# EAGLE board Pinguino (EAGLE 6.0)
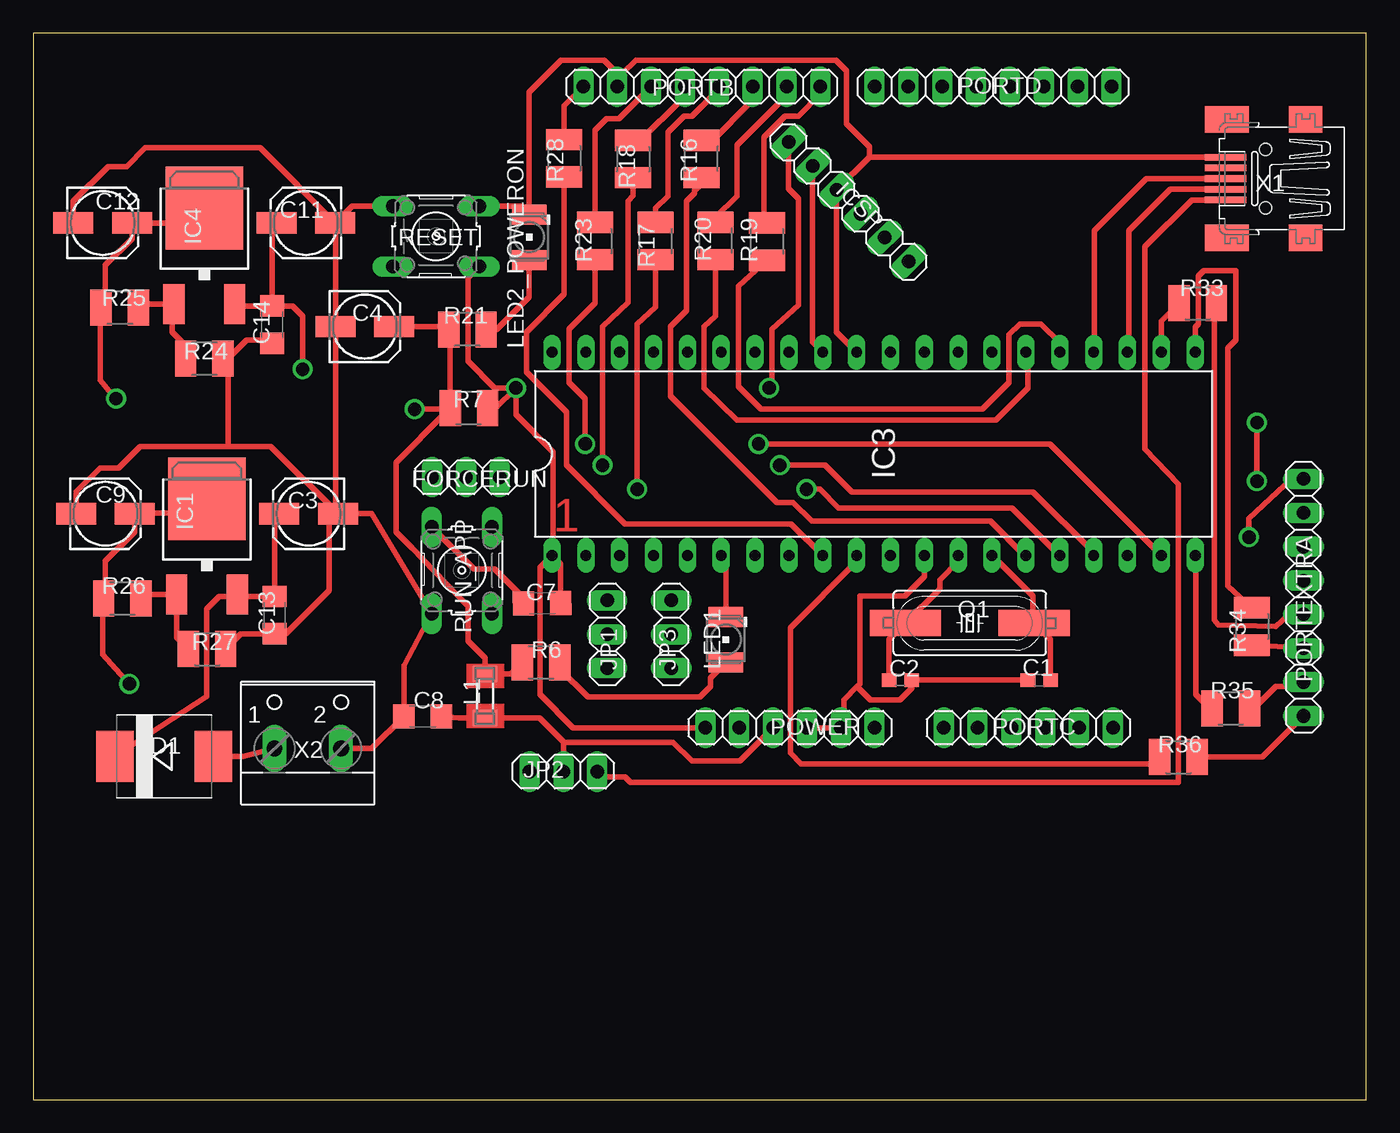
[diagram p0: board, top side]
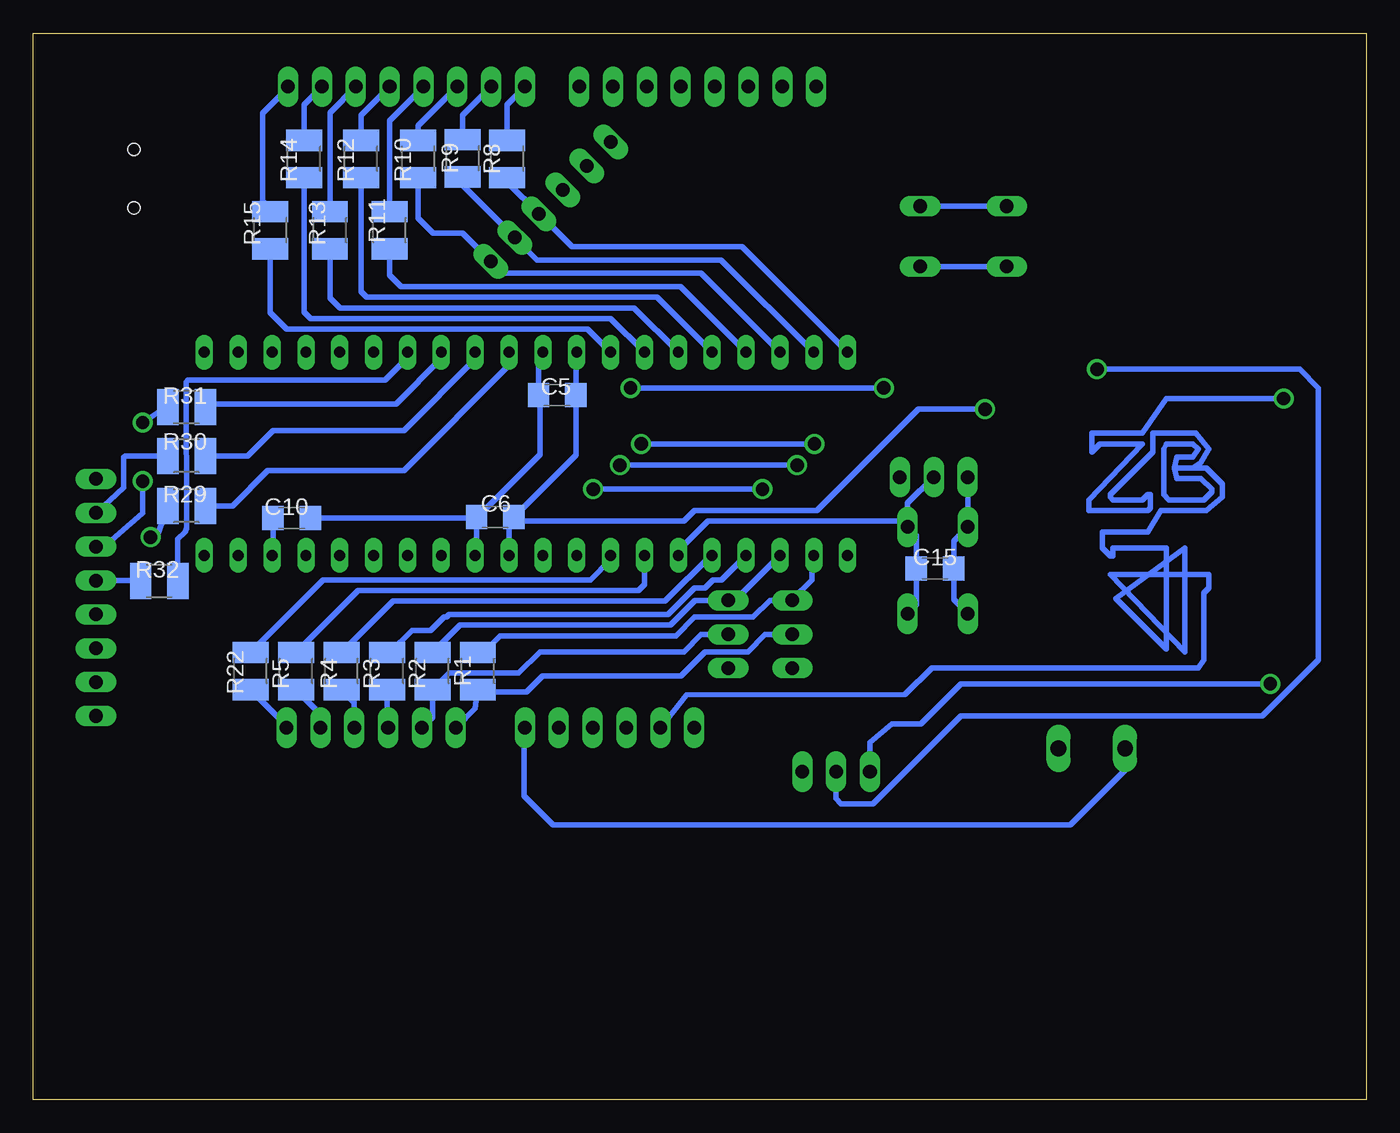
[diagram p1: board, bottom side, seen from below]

Size 100 x 80 mm. Coordinates in mm from the lower left corner, seen from the top.
Outline: 0,0 100,0 100,80 0,80 0,0
Copper layers (1*16): Top 0.035mm / dielectric 1.5mm / Bottom 0.035mm
Design rules: minimum track width 10mil, minimum drill 24mil, track to track 8mil, track to pad 8mil, pad to pad 8mil, via to via 8mil, smd to smd 8mil, copper to edge 40mil, drill to drill 8mil, minimum pad ring 10mil, minimum via ring 8mil, stop-mask expansion 4mil, vias tented up to drill 0mil, thermal gap 10mil

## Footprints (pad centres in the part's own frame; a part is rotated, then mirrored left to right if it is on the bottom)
C0603 = smd 1.1 x 1: 1 -0.85,0; 2 0.85,0
153CLV-0505 = smd 3 x 1.6: + 2.2,0; - -2.2,0
C1206 = smd 1.6 x 1.8: 1 -1.4,0; 2 1.4,0
SMC = smd 2.8 x 3.8: A 3.7,0; C -3.7,0
1X03 = drill 1.016 long: 1 -2.54,0; 2 0,0; 3 2.54,0
DPACK = smd 1.6 x 3: 1 -2.28,-4.8; 3 2.28,-4.8 | smd 5.8 x 6.2: 4 0,2.38
DIL40 = drill 0.813 long: 1 -24.13,-7.62; 2 -21.59,-7.62; 3 -19.05,-7.62; 4 -16.51,-7.62; 5 -13.97,-7.62; 6 -11.43,-7.62; 7 -8.89,-7.62; 8 -6.35,-7.62; 9 -3.81,-7.62; 10 -1.27,-7.62; 11 1.27,-7.62; 12 3.81,-7.62; 13 6.35,-7.62; 14 8.89,-7.62; 15 11.43,-7.62; 16 13.97,-7.62; 17 16.51,-7.62; 18 19.05,-7.62; 19 21.59,-7.62; 20 24.13,-7.62; 21 24.13,7.62; 22 21.59,7.62; 23 19.05,7.62; 24 16.51,7.62; 25 13.97,7.62; 26 11.43,7.62; 27 8.89,7.62; 28 6.35,7.62; 29 3.81,7.62; 30 1.27,7.62; 31 -1.27,7.62; 32 -3.81,7.62; 33 -6.35,7.62; 34 -8.89,7.62; 35 -11.43,7.62; 36 -13.97,7.62; 37 -16.51,7.62; 38 -19.05,7.62; 39 -21.59,7.62; 40 -24.13,7.62
1X06 = drill 1.016 long: 1 -6.35,0; 2 -3.81,0; 3 -1.27,0; 4 1.27,0; 5 3.81,0; 6 6.35,0
SM-1206 = smd 1.2 x 1.8: 1 -1.65,0; 2 1.65,0
PLCC2 = smd 2.6 x 1.5: A 0,1.7; C 0,-1.7
1X08 = drill 1.016 long: 1 -8.89,0; 2 -6.35,0; 3 -3.81,0; 4 -1.27,0; 5 1.27,0; 6 3.81,0; 7 6.35,0; 8 8.89,0
HC49UP = smd 5.334 x 1.93: 1 -4.826,0; 2 4.826,0
R1210 = smd 1.6 x 2.7: 1 -1.4,0; 2 1.4,0
B3F-10XX = drill 1.016 long: 1 -3.251,2.261; 2 3.251,2.261; 3 -3.251,-2.261; 4 3.251,-2.261
32005-201 = smd 3.1 x 0.5: 1 3,1.6; 2 3,0.8; 3 3,0; 4 3,-0.8; 5 3,-1.6 | smd 2.5 x 2: M1 -3,-4.45; M2 -3,4.45 | smd 3.3 x 2: M3 2.9,4.45; M4 2.9,-4.45 | hole 0.9: 0,2.2; 0,-2.2
W237-102 = drill 1.194 long: 1 -2.5,-1.27; 2 2.5,-1.27

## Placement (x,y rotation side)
C1  22pF  [C0603]  75.47,31.47 180 top
C2  22pF  [C0603]  65.05,31.47 0 top
C3  10uF  [153CLV-0505]  20.65,43.96 180 top
C4  10uF  [153CLV-0505]  24.87,58 0 top
C5  100nF  [C1206]  60.7,52.86 180 bottom
C6  100nF  [C1206]  65.35,43.72 0 bottom
C7  10nF  [C1206]  38.17,37.24 180.7 top
C8  100nF  [C1206]  29.21,28.76 0 top
C9  10uF  [153CLV-0505]  5.41,43.96 0 top
C10  220nF  [C1206]  80.62,43.64 180 bottom
C11  10uF  [153CLV-0505]  20.45,65.77 180 top
C12  10uF  [153CLV-0505]  5.21,65.77 0 top
C13  100nF  [C1206]  18.11,36.34 90 top
C14  100nF  [C1206]  17.91,58.15 90 top
C15  100nF  [C1206]  32.35,39.86 180 bottom
D1  MBRS320T3  [SMC]  9.82,25.75 0 top
FORCERUN  [1X03]  32.45,46.7 0 top
IC1  LD117ADT-TR  [DPACK]  13.03,42.69 0 top
IC3  PIC18F4550_40  [DIL40]  63.04,48.45 0 top
IC4  LD117ADT-TR  [DPACK]  12.83,64.5 0 top
ICSP  [1X06]  61.17,67.36 135.1 top
JP1  [1X03]  43.05,34.91 90 top
JP2  [1X03]  39.77,24.61 180 top
JP3  [1X03]  47.86,34.91 90 top
L1  300uH  [SM-1206]  33.88,30.27 270 top
LED1  LG_T679-E1F1-1  [PLCC2]  51.96,34.51 180 top
LED2_POWERON  LG_T679-E1F1-1  [PLCC2]  37.21,64.7 180 top
PORTB  [1X08]  50.16,76 180 top
PORTC  [1X06]  74.65,27.9 0 top
PORTD  [1X08]  72,76 0 top
PORTEXTRA  [1X08]  95.29,37.67 270 top
POWER  [1X06]  56.77,27.9 0 top
Q1  20MHz  [HC49UP]  70.26,35.75 0 top
R1  470  [R1210]  66.65,32.14 90 bottom
R2  470  [R1210]  70.06,32.14 90 bottom
R3  470  [R1210]  73.47,32.14 90 bottom
R4  470  [R1210]  76.88,32.14 90 bottom
R5  470  [R1210]  80.29,32.14 90 bottom
R6  470  [R1210]  38.09,32.8 0 top
R7  10k  [R1210]  32.68,51.88 180 top
R8  470  [R1210]  64.45,70.57 90 bottom
R9  470  [R1210]  67.79,70.62 90 bottom
R10  470  [R1210]  71.13,70.57 90 bottom
R11  470  [R1210]  73.27,65.22 90 bottom
R12  470  [R1210]  75.41,70.57 90 bottom
R13  470  [R1210]  77.75,65.22 90 bottom
R14  470  [R1210]  79.69,70.57 90 bottom
R15  470  [R1210]  82.23,65.22 90 bottom
R16  470  [R1210]  50.13,70.57 90 top
R17  470  [R1210]  46.67,64.42 270 top
R18  470  [R1210]  45.01,70.57 270 top
R19  470  [R1210]  55.05,64.37 90 top
R20  470  [R1210]  51.19,64.42 90 top
R21  470  [R1210]  32.57,57.77 180 top
R22  470  [R1210]  83.7,32.14 90 bottom
R23  470  [R1210]  42.15,64.42 270 top
R24  200  [R1210]  12.83,55.61 0 top
R25  120  [R1210]  6.48,59.42 0 top
R26  120  [R1210]  6.68,37.61 0 top
R27  360  [R1210]  13.03,33.8 0 top
R28  470  [R1210]  39.83,70.62 270 top
R29  470  [R1210]  88.5,44.55 180 bottom
R30  470  [R1210]  88.5,48.3 180 bottom
R31  470  [R1210]  88.5,51.95 180 bottom
R32  470  [R1210]  90.55,38.9 180 bottom
R33  470  [R1210]  87.36,59.75 0 top
R34  470  [R1210]  91.43,35.5 270 top
R35  470  [R1210]  89.84,29.35 0 top
R36  470  [R1210]  85.91,25.7 0 top
RESET  [B3F-10XX]  30.21,64.77 0 top
RUN_APP  [B3F-10XX]  32.15,39.71 270 top
X1  MINI-USB-32005-201  [32005-201]  92.45,69.1 180 top
X2  [W237-102]  20.59,27.61 0 top

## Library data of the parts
C1-C4 C9 C11 C12 R1-R36 = rcl
C5-C8 C10 C13-C15 = resistor
D1 = diode
FORCERUN ICSP JP1-JP3 PORTB PORTC PORTD PORTEXTRA POWER = pinhead
IC1 IC4 = v-reg
IC3 = microchip; MF: MICROCHIP; MPN: PIC18F4550-I/P; OC_FARNELL: 9321357; OC_NEWARK: 74K8623
L1 = inductor-neosid; OC_FARNELL: unknown; OC_NEWARK: unknown
LED1 LED2_POWERON = led; COLOR: green
Q1 = crystal; OC_FARNELL: unknown; OC_NEWARK: unknown
RESET RUN_APP = switch-omron; MPN: B3F-1000; OC_FARNELL: 176432; OC_NEWARK: 36M3542
X1 = con-cypressindustries; OC_FARNELL: unknown; OC_NEWARK: unknown
X2 = con-wago-500; MPN: 237-102; OC_FARNELL: unknown; OC_NEWARK: 70K9898

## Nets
3.3V: C12.+ IC4.4 POWER.2 R25.1
5V: C8.2 C11.+ C14.2 IC4.3 JP2.2 L1.2 POWER.3
AN0: JP1.2 PORTC.1 R1.1
AN1: JP3.2 PORTC.2 R2.1
AN2: PORTC.3 R3.1
AN3: PORTC.4 R4.1
AN4: PORTC.5 R5.1
AN5: PORTC.6 R22.1
AREF: PORTB.8 R28.1
D0: PORTD.1 R8.2
D1: PORTD.2 R9.2
D2: PORTD.3 R10.2
D3: PORTD.4 R11.2
D4: PORTD.5 R12.2
D5: PORTD.6 R13.2
D6: PORTD.7 R14.2
D7: PORTD.8 R15.2
D8: PORTB.1 R19.2
D9: PORTB.2 R20.2
D10: PORTB.3 R16.2
D11: PORTB.4 R17.1
D12: PORTB.5 R18.1
D13: PORTB.6 R23.1
GND: C1.2 C2.2 C3.- C4.- C5.2 C6.1 C7.2 C8.1 C9.- C10.1 C11.- C12.- C13.1 C14.1 C15.1 FORCERUN.1 IC3.12 IC3.31 ICSP.4 LED2_POWERON.C PORTB.7 POWER.4 POWER.5 R24.2 R27.2 RESET.1 RESET.2 RUN_APP.3 RUN_APP.4 X1.5 X2.2
N$1: C1.1 IC3.14 Q1.2
N$2: C2.1 IC3.13 Q1.1
N$3: LED1.A R6.2
N$4: C10.2 IC3.18
N$5: IC3.8 R22.2
N$6: IC3.2 JP1.3 R1.2
N$7: IC3.3 JP3.3 R2.2
N$8: IC3.4 R3.2
N$9: IC3.5 R4.2
N$10: IC3.7 R5.2
N$11: C15.2 FORCERUN.2 IC3.6 LED1.C RUN_APP.1 RUN_APP.2
N$12: IC3.25 R19.1
N$13: IC3.26 R20.1
N$14: IC3.15 R16.1
N$15: JP2.1 X1.1
N$16: IC3.37 R11.1
N$17: IC3.36 R12.1
N$18: IC3.35 R13.1
N$19: IC3.34 R14.1
N$20: IC3.33 R15.1
N$21: C9.+ IC1.4 JP2.3 R26.1
N$22: IC3.23 X1.2
N$23: IC3.24 X1.3
N$24: C3.+ C13.2 D1.C IC1.3
N$25: IC4.1 R24.1 R25.2
N$26: IC3.16 R17.2
N$27: PORTEXTRA.1 R29.2
N$28: IC3.17 R18.2
N$29: IC1.1 R26.2 R27.1
N$30: LED2_POWERON.A R21.1
N$31: IC3.19 R23.2
N$32: PORTEXTRA.4 R32.2
N$33: PORTEXTRA.3 R31.2
N$34: IC3.9 R28.2
N$35: PORTEXTRA.2 R30.2
N$36: PORTEXTRA.5 R33.2
N$37: PORTEXTRA.6 R34.2
N$38: PORTEXTRA.7 R35.2
N$39: PORTEXTRA.8 R36.2
N$40: IC3.10 R36.1
N$41: IC3.20 R35.1
N$42: IC3.21 R34.1
N$43: IC3.22 R33.1
N$44: IC3.27 R32.1
N$45: IC3.28 R31.1
N$46: IC3.29 R30.1
N$47: IC3.30 R29.1
PGC: IC3.39 ICSP.2 R9.1
PGD: IC3.40 ICSP.3 R8.1
PGM: IC3.38 ICSP.1 R10.1
RESET: C7.1 IC3.1 ICSP.6 POWER.1 R7.1 RESET.3 RESET.4
VCC: C4.+ C5.1 C6.2 IC3.11 IC3.32 ICSP.5 L1.1 R6.1 R7.2 R21.2
VIN: D1.A POWER.6 X2.1

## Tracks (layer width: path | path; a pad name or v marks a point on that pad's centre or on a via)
3.3V  (via drill 1)
  Top 0.406: IC4.4 11.72,65.77 C12.+ 7.41,64.61 5.4,62.6 5.4,59.74 R25.1 5,59.4 5,54 6,52.8 v6.2,52.6
  Bottom 0.406: v6.2,52.6 15,52.6 16.8,50 20.6,50 20.6,48.6 20,49.2 16.8,49.2 20.8,45 20.8,44.2 16.4,44.2 16.2,44.4 16.2,45.4 16.4,45.4 16.8,45 19,45 19.2,45.2 19.2,45.4 16,48.6 16,50 12.8,50 11.8,48.8 12.4,47.8 13,47.4 | 13,47.4 14.4,47.4 | 14.4,47.4 14.2,48.2 13,48.2 12.6,48.8 13,49.2 15,49.2 15.2,48.8 15.2,45.4 14.8,45 12.2,45 11.6,45.6 11.6,45.8 12.4,46.6 14.2,46.6 14.4,47.4 | 13,47.4 12,47.4 10.8,46.2 10.8,45.2 12,44.2 15.4,44.2 16.4,42.6 19.8,42.6 19.8,41.4 19.2,40.8 19,40.8 19,41.4 15,41.4 15,33.8 18.8,37.6 13.6,41.4 13.6,33.6 19.2,39.4 11.8,39.4 11.8,38.4 12.2,38 12.2,33 12.6,32.4 32.6,32.4 34.6,30.4 51,30.34 POWER.2
5V  (via drill 1)
  Top 0.406: C14.2 17.91,65.11 18,65.2 18,65.52 C11.+ | C14.2 15.26,59.55 IC4.3 | C14.2 19.45,59.55 20.2,58.8 v20.2,54.8 | 39.8,26.8 37.98,28.62 L1.2 31.95,28.62 C8.2 | 39.8,26.8 48,26.8 49.4,25.4 53,25.4 POWER.3 | JP2.2 39.77,26.77 39.8,26.8
  Bottom 0.406: JP2.2 39.8,24.58 39.8,22.6 39.4,22.2 37,22.2 30.4,28.8 7.8,28.8 3.6,33 3.6,53.4 5,54.8 v20.2,54.8
AN0
  Bottom 0.406: PORTC.1 66.85,29.35 R1.1 66.51,30.6 63,30.6 61.8,31.8 51.4,31.8 49.6,33.6 46.4,33.6 45.09,34.91 JP1.2
AN1
  Bottom 0.406: PORTC.2 70.06,28.68 R2.1 68.8,32 63.6,32 62,33.6 51.2,33.6 49.89,34.91 JP3.2
AN2
  Bottom 0.406: R3.1 73.47,27.99 PORTC.3
AN3
  Bottom 0.406: PORTC.4 75.92,29.78 R4.1
AN4
  Bottom 0.406: PORTC.5 78.46,28.91 R5.1
AN5
  Bottom 0.406: PORTC.6 81,28.04 R22.1
AREF
  Top 0.406: R28.1 39.83,74.56 PORTB.8
D0
  Bottom 0.406: R8.2 64.45,74.66 PORTD.1
D1
  Bottom 0.406: R9.2 67.79,73.86 PORTD.2
D2
  Bottom 0.406: R10.2 71.13,73.06 PORTD.3
D3
  Bottom 0.406: R11.2 73.27,73.46 PORTD.4
D4
  Bottom 0.406: R12.2 75.41,73.86 PORTD.5
D5
  Bottom 0.406: R13.2 77.75,74.06 PORTD.6
D6
  Bottom 0.406: R14.2 79.69,74.66 PORTD.7
D7
  Bottom 0.406: PORTD.8 80.89,75.91 82.8,74 82.8,67.4 | 82.8,67.4 82.8,67.2 82.6,67 | R15.2 82.23,66.83 82.8,67.4
D8
  Top 0.406: PORTB.1 59.05,75.45 57.4,73.8 56.4,73.8 54.8,72.2 54.8,66.22 R19.2
D9
  Top 0.406: R20.2 51.19,66.19 52.8,67.8 52.8,71.6 56.4,75.2 56.4,75.89 PORTB.2
D10
  Top 0.406: PORTB.3 53.97,74.97 50.8,71.8 50.3,71.8 R16.2
D11
  Top 0.406: R17.1 46.67,66.87 47.6,67.8 47.6,72.6 48.8,73.8 49.4,73.8 51.2,75.57 PORTB.4
D12
  Top 0.406: R18.1 45.57,71.97 48.6,75 48.6,75.71 PORTB.5
D13
  Top 0.406: R23.1 42.15,72.75 43,73.6 43.95,73.6 PORTB.6
GND
  Top 0.406: R27.2 15.57,34.94 C13.1 18.94,34.94 22.2,38.2 22.2,43.31 C3.- | C9.- 3.21,45.61 5,47.4 6.4,47.4 8,49 14.6,49 | 14.6,49 17.81,49 C3.- | C12.- 3.01,67.41 5.6,70 7,70 8.4,71.4 17.02,71.4 C11.- | C14.1 17.66,57 16,57 14.61,55.61 R24.2 14.6,55.24 14.6,49 | C11.- 22.67,65.75 C4.- 22.67,44.14 C3.- | IC3.31 60.27,57.57 ICSP.4 62.71,70.7 | C1.2 C2.2 65.9,30.9 65,30 62.8,30 61.8,31 | IC3.12 66.85,39.25 65.4,37.8 62,37.8 62,31.2 61.8,31 | 61.8,31 60.8,30 60.8,28.12 POWER.5 POWER.4 | 62.71,70.7 X1.5 | 62.71,70.7 62.71,71.49 61,73.2 61,77.2 60.2,78 45.2,78 44.19,76.99 43.81,76.99 | C7.2 36.77,37.63 34.6,39.8 33.05,39.8 RUN_APP.3 | RESET.2 36.58,67.03 LED2_POWERON.C 37.2,75.6 39.6,78 42.8,78 43.81,76.99 | C3.- 25.39,43.96 RUN_APP.4 27.81,32.58 C8.1 25.39,26.34 X2.2 | RESET.1 23.91,67.03 C11.- | 43.81,76.99 PORTB.7
  Bottom 0.406: IC3.31 62.1,55.74 C5.2 62,52.76 62,48.4 66.68,43.72 C6.1 | C6.1 66.75,40.93 IC3.12 | C10.1 66.83,43.64 C6.1 | FORCERUN.1 29.89,46.68 RUN_APP.3 30.95,41.9 C15.1 30.95,37.52 RUN_APP.4 | RESET.1 RESET.2
N$1
  Top 0.406: C1.1 76.32,34.52 Q1.2 75,35.84 75,37.8 71.97,40.83 IC3.14
N$2
  Top 0.406: C2.1 64.2,34.52 Q1.1 68,38.32 68,39 69.39,40.39 IC3.13
N$3
  Top 0.406: R6.2 39.49,32.31 41.6,30.2 50,30.2 50.8,31 50.8,31.65 LED1.A
N$4
  Bottom 0.406: C10.2 82.02,40.9 IC3.18
N$5
  Bottom 0.406: IC3.8 56.69,40.51 58.2,39 78.24,39 R22.2
N$6
  Bottom 0.406: IC3.2 41.6,40.68 41.6,39 43.05,37.55 JP1.3 44.75,37.45 46,36.2 50.4,36.2 51.8,34.8 65,34.8 66.4,33.4 66.4,33.54 R1.2 66.71,33.6 65.6,33.6
N$7
  Bottom 0.406: IC3.3 47.37,37.45 JP3.3 50.35,37.45 52.2,35.6 68,35.6 R2.2
N$8
  Bottom 0.406: R3.2 73.26,33.54 71.6,35.2 70.2,35.2 69.2,36.2 69,36.2 68.8,36.4 52.4,36.4 50.4,38.4 49.6,38.4 49,39 48.36,39 IC3.4
N$9
  Bottom 0.406: IC3.5 49.17,40.83 52.6,37.4 73.02,37.4 R4.2
N$10
  Bottom 0.406: IC3.7 54.15,38.65 54.6,38.2 75.63,38.2 R5.2
N$11
  Top 0.406: LED1.C 51.96,40.48 IC3.6
  Bottom 0.406: IC3.6 51.61,41.19 49.4,43.4 34.85,43.4 RUN_APP.1 | RUN_APP.1 34.41,44.74 FORCERUN.2 | RUN_APP.1 33.75,42.3 C15.2 33.75,37.12 RUN_APP.2
N$12
  Top 0.406: IC3.25 77.01,56.79 75.6,58.2 74,58.2 73.2,57.4 73.2,53.8 71.2,51.8 54.6,51.8 52.9,53.5 52.9,61.02 R19.1
N$13
  Top 0.406: R20.1 51.19,58.79 50.3,58 50.3,53.4 52.8,51 72.2,51 74.6,53.4 74.6,55.94 IC3.26
N$14
  Top 0.406: R16.1 50.13,68.73 49.6,68.2 49.6,68 49,67.4 49,59.2 47.8,58 47.8,52.8 55.8,44.8 57,44.8 58.4,43.4 71.8,43.4 74.37,40.83 IC3.15
N$15
  Top 0.406: X1.1 86.9,67.5 83.4,64 83.4,48.8 85.9,46.2 85.9,23.8 44.8,23.8 44.4,24.2 42.72,24.2 JP2.1
N$16
  Bottom 0.406: R11.1 73.27,61.87 72.4,61 51.46,61 IC3.37
N$17
  Bottom 0.406: R12.1 75.41,60.61 75,60.2 53.2,60.2 IC3.36
N$18
  Bottom 0.406: R13.1 77.75,60.15 77,59.4 54.94,59.4 IC3.35
N$19
  Bottom 0.406: R14.1 79.69,59.09 79.2,58.6 56.68,58.6 IC3.34
N$20
  Bottom 0.406: R15.1 82.23,59.03 81,57.8 58.42,57.8 IC3.33
N$21  (via drill 1)
  Top 0.406: IC1.4 12.47,45.07 11.4,44 7.65,44 C9.+ 7.61,43.99 7.6,44 7.6,42.6 5.4,40.4 5.4,37.73 R26.1 5.2,37.6 5.2,33.4 v7.2,31.2
  Bottom 0.406: 37,24.6 JP2.3 37.22,26.8 35.6,28.2 33.4,28.2 30.4,31.2 v7.2,31.2
N$22
  Top 0.406: X1.2 85.3,68.3 82.2,65.2 82.2,56.18 IC3.23
N$23
  Top 0.406: X1.3 83.5,69.1 79.6,65.2 79.6,56.12 IC3.24
N$24
  Top 0.406: 15.46,37.74 C13.2 18.11,43.62 C3.+ | 15.46,37.74 IC1.3 | 15.46,37.74 13.94,37.74 13,36.8 13,30.23 D1.C
N$25
  Top 0.406: R24.1 11.43,56.57 10.4,57.6 10.4,59.55 IC4.1 8.16,59.7 R25.2
N$26  (via drill 1)
  Top 0.406: IC3.16 76.97,40.83 73.4,44.4 60.4,44.4 59,45.8 v58,45.8 | R17.2 46.67,59.47 45.3,58.2 v45.3,45.8
  Bottom 0.406: v45.3,45.8 v58,45.8
N$27  (via drill 1)
  Top 0.406: v91.2,42.2 91.2,43.6 94.4,46.6 95.2,46.6 PORTEXTRA.1
  Bottom 0.406: 91.1,42.1 90.6,42.6 R29.2 | 91.1,42.1 91.2,42 | v91.2,42.2 91.1,42.1
N$28  (via drill 1)
  Top 0.406: R18.2 45.01,67.81 44.6,67.4 44.6,59.8 42.7,58 v42.7,47.6 | IC3.17 79.55,41.05 75,45.6 61.4,45.6 59.4,47.6 v56,47.6
  Bottom 0.406: v42.7,47.6 v56,47.6
N$29
  Top 0.406: R26.2 8.36,37.89 IC1.1 10.75,34.68 R27.1
N$30
  Top 0.406: R21.1 34.77,57.77 37.2,60.2 LED2_POWERON.A
N$31  (via drill 1)
  Top 0.406: R23.2 42.15,59.75 40.2,57.8 40.2,53.8 41.4,52.6 v41.4,49.2 | v54.4,49.2 76.26,49.2 IC3.19
  Bottom 0.406: v41.4,49.2 v54.4,49.2
N$32
  Bottom 0.406: PORTEXTRA.4 91.99,38.94 R32.2
N$33  (via drill 1)
  Top 0.406: v91.8,46.4 v91.8,50.8
  Bottom 0.406: v91.8,50.8 90.6,51.6 R31.2 | v91.8,46.4 91.8,44 95.01,41.2 PORTEXTRA.3
N$34
  Top 0.406: R28.2 39.83,60.43 37,57.6 37,54.6 40,51.6 40,47.6 44.4,43.2 56.86,43.2 IC3.9
N$35
  Bottom 0.406: R30.2 93.1,48.3 93.2,48.2 93.2,45.91 PORTEXTRA.2
N$36
  Top 0.406: PORTEXTRA.5 94.2,36.4 93.2,35.5 88.9,35.6 88.6,36 88.6,59.59 R33.2
N$37
  Top 0.406: R34.2 95.25,33.9 PORTEXTRA.6
N$38
  Top 0.406: R35.2 91.55,29.35 93.2,31 94.97,31 PORTEXTRA.7
N$39
  Top 0.406: R36.2 92.21,25.7 PORTEXTRA.8
N$40
  Top 0.406: IC3.10 61.77,40.37 56.8,35.4 56.8,26 57.6,25.2 84.01,25.2 R36.1
N$41
  Top 0.406: R35.1 88.25,29.35 87.2,30.4 87.2,40.8 IC3.20
N$42
  Top 0.406: IC3.21 87.17,57.97 87.4,58.2 87.4,61.8 87.8,62.2 90.2,62.2 90.2,57 89.6,56.4 89.6,38.53 R34.1
N$43
  Top 0.406: IC3.22 84.63,58.42 R33.1
N$44
  Bottom 0.406: IC3.27 71.93,55.67 73.6,54 88.4,54 88.55,53.85 88.5,42.9 88.6,42.6 89.15,42.05 R32.1
N$45
  Bottom 0.406: IC3.28 69.39,55.61 72.8,52.2 86.83,52.2 R31.1
N$46
  Bottom 0.406: IC3.29 66.85,55.55 72.2,50.2 82,50.2 83.9,48.3 R30.1
N$47
  Bottom 0.406: IC3.30 64.31,55.09 72.2,47.2 82.4,47.2 85.05,44.55 R29.1
PGC
  Bottom 0.406: R9.1 67.79,68.59 ICSP.2 62.2,63 48.4,63 41.47,56.07 IC3.39
PGD
  Bottom 0.406: R8.1 64.45,68.84 ICSP.3 59.6,64 46.84,64 IC3.40
PGM
  Bottom 0.406: R10.1 71.13,66.13 70,65 67.79,65 ICSP.1 65.48,62.88 64.6,62 49.92,62 IC3.38
RESET  (via drill 1)
  Top 0.406: ICSP.6 56.67,68.33 57.4,67.6 57.4,59.6 55.4,57.8 55.4,53.4 v55.2,53.4 | v36.2,53.4 36.2,51.4 39,48.6 39,41 IC3.1 | POWER.1 40.5,27.9 38,30.4 38,39.92 IC3.1 | C7.1 39.57,40.17 IC3.1 | R7.1 34.68,51.88 v36.2,53.4 | v36.2,53.4 34.6,53.4 32.6,55.4 32.6,61.65 RESET.4
  Bottom 0.406: v36.2,53.4 v55.2,53.4 | RESET.4 RESET.3
VCC  (via drill 1)
  Top 0.406: ICSP.5 58.47,56.83 IC3.32 | R6.1 35.81,31.92 L1.1 33.88,33.12 32.6,34.4 32.6,37 28.4,41.4 27.2,42.6 27.2,47.8 30.9,51.5 | 30.9,51.5 R7.2 31.28,57.66 R21.2 30.94,58 C4.+ | v28.6,51.8 30.6,51.8 30.9,51.5
  Bottom 0.406: IC3.32 59.3,56 C5.1 59.3,48.37 C6.2 | IC3.11 64.31,43.36 C6.2 | v28.6,51.8 33.6,51.8 41.2,44.2 50.4,44.2 51.2,43.4 63.63,43.4 C6.2
VIN
  Top 0.406: X2.1 15.73,25.74 D1.A
  Bottom 0.406: X2.1 18.09,24.71 22.2,20.6 61,20.6 63.2,22.8 63.2,27.82 POWER.6
(copper drawn outside any net)
  shapes: Top area x2

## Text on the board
Top: 1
